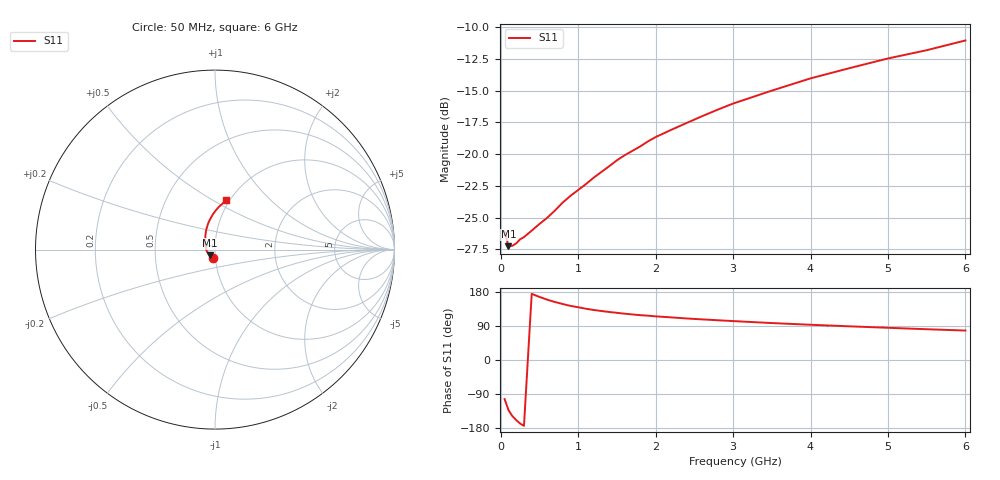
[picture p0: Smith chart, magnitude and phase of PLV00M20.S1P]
! Infineon Technologies  Discrete & RF Semiconductors
! BAR 64-04W /-05W /-06W
! Si PIN Diode in SOT323
! IF = 0.2 mA
! S-Parameters:  October  2008
# GHz  S  MA  R  50
!  f  S11
! GHz  MAG  ANG
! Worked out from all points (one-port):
!   34 points, 50 MHz to 6 GHz, reference 50 ohm
!   lowest |S11| = -27.3 dB at 100 MHz (marker M1), VSWR 1.09, Z = 47.1 - j3.03 ohm
!   |S11| at or under -10 dB: start of sweep to end of sweep
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0.05  0.04962 -103.1
0.1  0.04337 -132.2
0.15  0.04352 -148.1
0.2  0.04448 -158.5
0.25  0.04615 -167.7
0.3  0.0471 -173.8
0.4  0.04994 174.6
0.5  0.05306 166.4
0.6  0.05612 159.2
0.7  0.05994 153.1
0.8  0.06442 147.7
0.9  0.06845 142.8
1.1  0.0762 135.3
1.2  0.08077 132.0
1.5  0.09457 124.5
1.6  0.099 122.2
1.8  0.1072 118.4
1.9  0.1122 117.0
2  0.1167 115.2
2.4  0.1327 109.6
2.8  0.1497 104.9
3  0.1583 102.7
3.5  0.178 97.5
4  0.1989 93.0
4.5  0.2182 88.9
5  0.2384 85.0
5.5  0.2569 81.2
6  0.2807 77.7
